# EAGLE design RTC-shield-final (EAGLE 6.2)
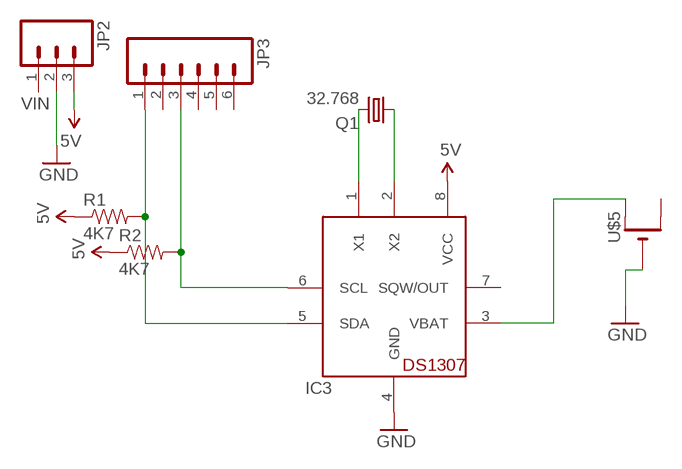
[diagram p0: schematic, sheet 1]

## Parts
IC3  DS1307  [DIL08]
JP2  M03PTH  [1X03]
JP3  M06SIP  [1X06]
Q1  32.768  CRYTALTC38H  [TC38H]
R1  4K7  RESISTORAXIAL-0.3  [AXIAL-0.3]
R2  4K7  RESISTORAXIAL-0.3  [AXIAL-0.3]
U$5  CR1220THM-PAD  [CR1220-THM-PAD]

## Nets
5V: IC3.8(VCC) JP2.3 R1.P$1 R2.P$1
GND: IC3.4(GND) JP2.2 U$5.-
N$1: IC3.3(VBAT) U$5.+1(+)
N$3: IC3.6(SCL) JP3.3 R2.P$2
N$4: IC3.5(SDA) JP3.1 R1.P$2
N$14: IC3.1(X1) Q1.2
N$15: IC3.2(X2) Q1.1
Unconnected: IC3.7(SQW/OUT) JP2.1 JP3.2 JP3.4 JP3.5 JP3.6 U$5.+2(+1)

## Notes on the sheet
- VIN

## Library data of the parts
IC3 = adafruit:DS1307: DS1307 Real time clock (RTC) with battery backup ability. Talk to it via i2c
JP2 = SparkFun:M03: Header 3 Standard 3-pin 0.1" header. Use with straight break away headers (SKU : PRT-00116), right angle break away headers (PRT-00553), swiss pins (PRT-00743), machine pins (PRT-00117), and female headers (PRT-00115). Molex polarized connector foot print use with SKU : PRT-08232 with associated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
JP3 = SparkFun:M06: Header 6 Standard 6-pin 0.1" header. Use with straight break away headers (SKU : PRT-00116), right angle break away headers (PRT-00553), swiss pins (PRT-00743), machine pins (PRT-00117), and female headers (PRT-00115). Molex polarized connector foot print use with SKU : PRT-08094 with associated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
Q1 = crystal:CRYTAL: CRYSTAL
R1 R2 = SparkFun:RESISTOR: Resistor
U$5 = adafruit:CR1220: CR1216/CR1220/CR1225 12mm 3V lithium coin cell Great for battery packup. Both SMT and THM holders. Note the THM package has the ground pads on both sides of the PCB so that the masks are the same - this reduces the cost

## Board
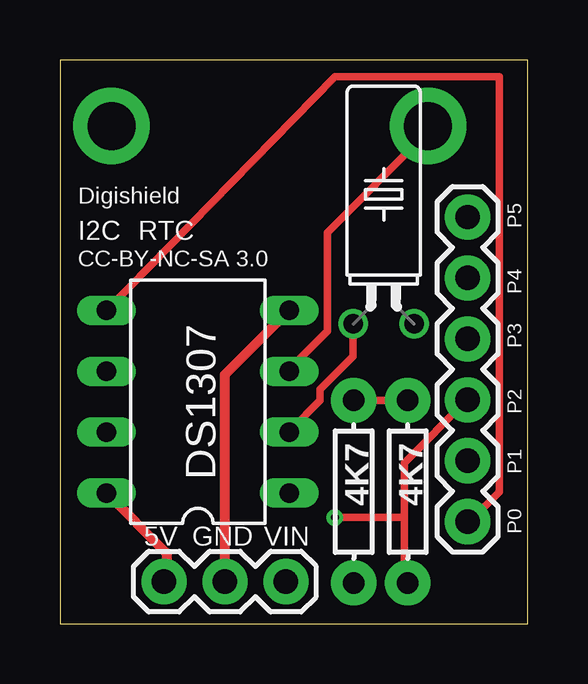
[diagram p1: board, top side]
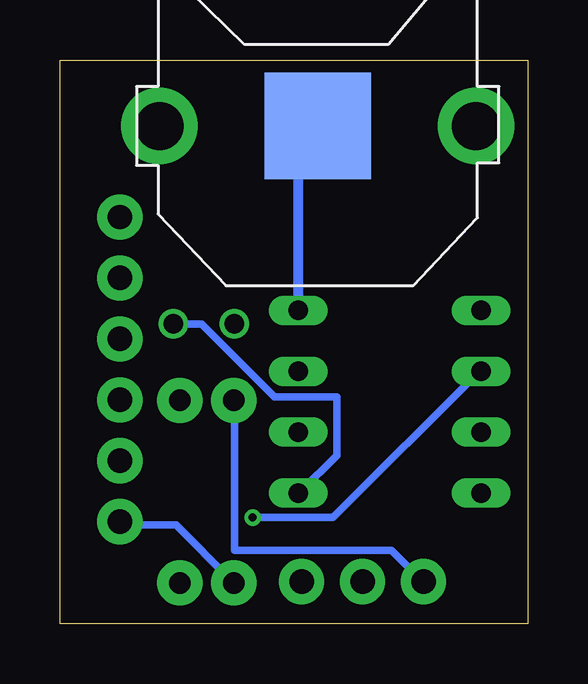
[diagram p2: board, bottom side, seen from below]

Size 19.5 x 23.5 mm. Coordinates in mm from the lower left corner, seen from the top.
Outline: 0,23.5 0,0 19.5,0 19.5,23.5 0,23.5
Copper layers (1*16): Top 0.0356mm / dielectric 1.5011mm / Bottom 0.0356mm
Design rules: minimum track width 12mil, minimum drill 13mil, track to track 8mil, track to pad 8mil, pad to pad 8mil, via to via 8mil, smd to smd 8mil, copper to edge 15mil, drill to drill 12mil, minimum pad ring 7mil, minimum via ring 7mil, stop-mask expansion 4mil, vias tented up to drill 0mil, thermal gap 10mil

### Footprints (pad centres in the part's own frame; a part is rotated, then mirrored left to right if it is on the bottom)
DIL08 = drill 0.813 long: 1 -3.81,-3.81; 2 -1.27,-3.81; 3 1.27,-3.81; 4 3.81,-3.81; 5 3.81,3.81; 6 1.27,3.81; 7 -1.27,3.81; 8 -3.81,3.81
1X03 = drill 1.016 pad 1.88: 1 0,0; 2 2.54,0; 3 5.08,0
1X06 = drill 1.016 pad 1.88: 1 0,0; 2 2.54,0; 3 5.08,0; 4 7.62,0; 5 10.16,0; 6 12.7,0
TC38H = drill 0.813: 1 -1.27,0; 2 1.27,0
AXIAL-0.3 = drill 0.9 pad 1.88: P$1 -3.81,0; P$2 3.81,0
CR1220-THM-PAD = drill 2 pad 3.175: +1 -6.604,0; +2 6.604,0 | smd 4.445 x 4.445: - 0,0

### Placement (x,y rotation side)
IC3  5.75,9.25 90 top
JP2  9.42,1.75 180 top
JP3  17,4.25 90 top
Q1  13.5,12.5 0 top
R1  12.25,5.5 270 top
R2  14.5,5.5 270 top
U$5  8.75,20.75 0 bottom

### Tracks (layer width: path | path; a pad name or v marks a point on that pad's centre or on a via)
5V
  Top 0.305: R1.P$1 12.38,9.3 14.36,9.3 R2.P$1
  Top 0.406: IC3.8 4.45,2.93 4.45,1.86 JP2.3
  Bottom 0.305: R1.P$1 12.22,9.3 12.22,3.05 5.67,3.05 4.45,1.83 JP2.3
GND
  Top 0.406: JP2.2 6.88,10.38 IC3.4
  Bottom 0.406: IC3.4 9.56,19.69 U$5.-
N$1
  Top 0.305: IC3.3 9.63,10.67 11.16,12.19 11.16,16.31 15.27,20.42 U$5.+1
N$3  (via drill 0.33)
  Top 0.305: 14.36,4.42 v11.46,4.42 | 14.36,4.42 14.36,1.83 R2.P$2 | 14.36,4.42 14.36,6.71 16.95,9.3 JP3.3
  Bottom 0.305: v11.46,4.42 8.11,4.42 2.01,10.52 IC3.6
N$4
  Top 0.305: IC3.5 2.01,13.11 11.46,22.8 18.32,22.8 18.32,5.49 17.1,4.27 JP3.1
  Bottom 0.305: R1.P$2 12.38,1.83 14.66,4.12 16.95,4.12 JP3.1
N$14
  Bottom 0.305: IC3.1 9.48,5.49 7.96,7.01 7.96,9.45 10.55,9.45 13.59,12.5 14.66,12.5 Q1.2
N$15
  Top 0.305: IC3.2 9.63,8.08 10.85,9.3 10.85,9.75 12.22,11.12 Q1.1

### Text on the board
tPlace: Digishield | I2C | RTC | CC-BY-NC-SA 3.0 | DS1307 | 5V | GND | VIN
tNames: P5 | P4 | P3 | P2 | P1 | P0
